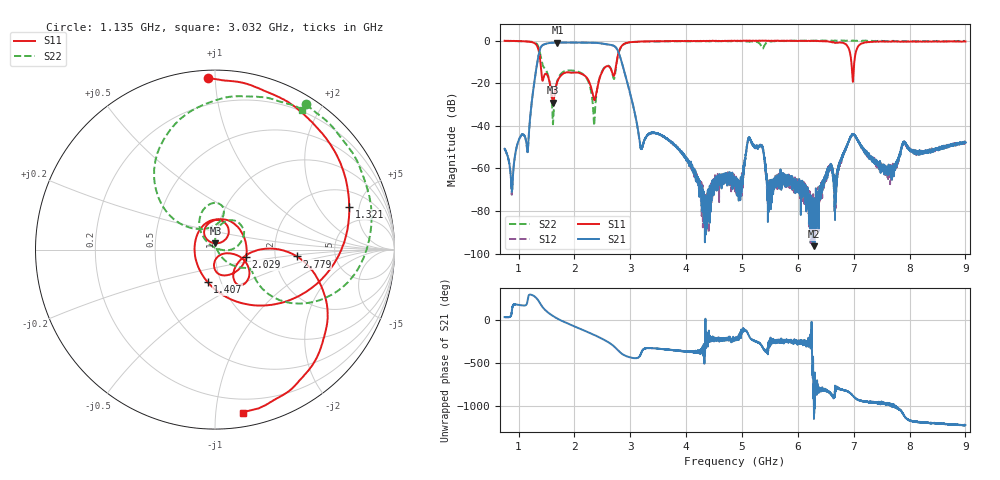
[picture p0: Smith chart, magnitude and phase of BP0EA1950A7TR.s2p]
!Agilent Technologies,E8358A,US41080443,A.07.50.56
!Agilent E8358A: A.07.50.56
!Date: Friday, November 20, 2015 11:14:12
!Correction: S11(Full 2 Port(1,2))
!S21(Full 2 Port(1,2))
!S12(Full 2 Port(1,2))
!S22(Full 2 Port(1,2))
!S2P File: Measurements: S11, S21, S12, S22:
# Hz S  dB  R 50
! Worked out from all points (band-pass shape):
!   6401 points, 750 MHz to 9 GHz, reference 50 ohm
!   highest |S21| = -0.94 dB at 1.696 GHz (marker M1); lowest = -96.5 dB at 6.281 GHz (marker M2)
!   |S21| within 3 dB of the highest: 1.387 GHz to 2.76 GHz (1.373 GHz wide, 66.2 % of centre)
!   lowest |S11| = -29.1 dB at 1.616 GHz (marker M3), VSWR 1.07, Z = 50.2 + j3.5 ohm
!   |S11| at or under -10 dB: 1.39 GHz to 2.754 GHz (1.364 GHz wide, 65.8 % of centre); 6.958 GHz to 7.012 GHz (53.48 MHz wide, 0.766 % of centre)
!   |S22| runs from -40.0 to 0.0 dB; largest |S21 - S12| = 0.0065
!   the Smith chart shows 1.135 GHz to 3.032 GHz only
!   S11 on the Smith chart (normalised r, x): 1.135 GHz: 0.04, +0.96; 1.321 GHz: 3.16, +3.96; 1.407 GHz: 0.86, -0.32; 2.029 GHz: 1.41, -0.12; 2.779 GHz: 2.66, -0.26; 3.032 GHz: 0.10, -1.18
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7.5e8  -0.11 141.0  -50.79 38.8  -50.75 38.8  -0.21 114.0
1.13543e9  -0.40 92.5  -47.30 -178.2  -47.37 -177.8  -0.40 57.9
1.321055e9  -2.10 17.8  -12.54 -98.4  -12.58 -98.3  -1.47 0.0
1.407422e9  -14.66 -103.0  -2.78 177.6  -2.81 177.6  -8.93 -39.8
1.61625e9  -29.12 85.4  -0.98 52.4  -1.03 52.4  -39.29 24.8
1.696172e9  -19.15 123.4  -0.94 21.5  -0.98 21.5  -18.71 82.5
2.02875e9  -14.99 -13.3  -0.97 -78.3  -1.01 -78.3  -14.28 33.7
2.12543e9  -15.57 -52.1  -0.96 -104.6  -1.01 -104.6  -15.29 23.9
2.420625e9  -20.86 -13.8  -1.14 169.7  -1.18 169.7  -20.70 133.3
2.778984e9  -6.79 -4.8  -4.88 9.7  -4.95 9.7  -7.17 136.7
3.031641e9  -0.71 -80.3  -28.38 -78.7  -28.37 -79.1  -0.75 58.2
3.19793e9  -0.44 -102.0  -50.86 -18.4  -50.72 -19.5  -0.55 34.7
3.500859e9  -0.33 -128.2  -43.72 28.5  -43.86 28.5  -0.38 4.1
4.350352e9  -0.23 -168.3  -76.62 90.9  -72.55 -159.3  -0.36 -65.2
4.875e9  -0.13 178.1  -64.99 154.7  -65.98 146.2  -0.27 -99.4
5.143125e9  -0.06 -173.5  -46.17 158.2  -46.15 160.2  -0.50 -125.5
5.492461e9  -0.15 -172.8  -68.13 99.5  -72.62 96.3  -0.45 -130.6
6.25043e9  -0.13 -171.2  -77.42 173.0  -79.30 108.7  -0.12 -154.4
6.281367e9  -0.22 -171.1  -96.49 159.3  -87.68 139.5  -0.04 -155.6
6.977461e9  -17.23 157.3  -44.17 -157.6  -44.29 -158.0  -0.04 -162.5
7.625859e9  -0.51 178.1  -58.16 94.6  -62.12 109.7  -0.30 -174.2
9e9  -0.46 123.2  -47.80 -148.8  -47.79 -152.1  -0.20 127.1
